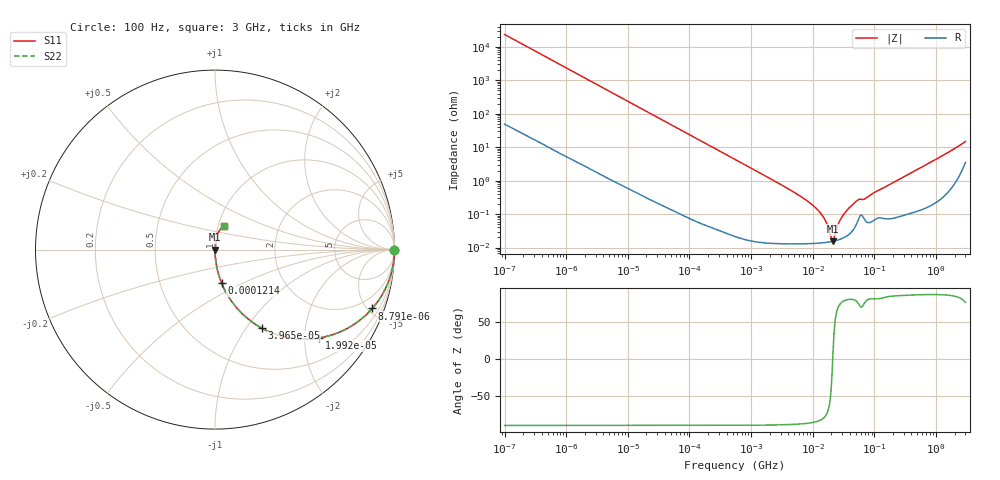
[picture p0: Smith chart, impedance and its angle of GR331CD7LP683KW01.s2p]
!Murata Part Number: GR331CD7LP683KW01
!These Parameters are Measured in Series Mode Connection
!Data Generated on Jan 08, 2026
!  o--ll--o
!Port1  Port2
!  o------o
!Operation Temp=25[degC], DC Bias Voltage=0[V]
!Freq. Start=100[Hz] Stop=3[GHz] 401[Steps]
# Hz S RI R 50
!Freq.(Hz) S11(Real) S11(Imag) S21(Real) S21(Imag) S12(Real) S12(Imag) S22(Real) S22(Imag)
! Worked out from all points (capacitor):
!   401 points, 100 Hz to 3 GHz, reference 50 ohm
!   read as one part in series: C = 68.2 nF near 109 Hz
!   lowest |Z| = 15.5 mohm at 21.25 MHz (marker M1)
!   series resonance near 21.1 MHz, so ESL is about 830 pH
!   S11 on the Smith chart (normalised r, x): 100 Hz: open; 8.791 kHz: 1.01, -5.34; 19.92 kHz: 1.01, -2.36; 39.66 kHz: 1.00, -1.19; 121.4 kHz: 1.00, -0.39; 3 GHz: 1.07, +0.28
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100  1 -0.00429  2.73e-05 0.00429  2.73e-05 0.00429  1 -0.00429
1788  0.994 -0.0759  0.00597 0.0759  0.00597 0.0759  0.994 -0.0759
8791  0.8763 -0.328  0.1237 0.328  0.1237 0.328  0.8763 -0.328
19917  0.5818 -0.492  0.4182 0.492  0.4182 0.492  0.5818 -0.492
31977  0.3514 -0.476  0.6486 0.476  0.6486 0.476  0.3514 -0.476
39655  0.2609 -0.4377  0.7391 0.4377  0.7391 0.4377  0.2609 -0.4377
66468  0.1122 -0.3142  0.8878 0.3142  0.8878 0.3142  0.1122 -0.3142
121426  0.0369 -0.1868  0.9631 0.1868  0.9631 0.1868  0.0369 -0.1868
547723  0.00207 -0.043  0.9979 0.043  0.9979 0.043  0.00207 -0.043
4141163  0.000159 -0.00549  0.9998 0.00549  0.9998 0.00549  0.000159 -0.00549
9794414  0.000135 -0.0019  0.9999 0.0019  0.9999 0.0019  0.000135 -0.0019
1.506283e7  0.00014 -0.000772  0.9999 0.000772  0.9999 0.000772  0.00014 -0.000772
1.713898e7  0.000144 -0.000471  0.9999 0.000471  0.9999 0.000471  0.000144 -0.000471
1.950129e7  0.00015 -0.000178  0.9999 0.000178  0.9999 0.000178  0.00015 -0.000178
2.12544e7  0.000154 1.66e-05  0.9998 -1.66e-05  0.9998 -1.66e-05  0.000154 1.66e-05
2.21892e7  0.000157 0.000114  0.9998 -0.000114  0.9998 -0.000114  0.000157 0.000114
2.999103e7  0.000188 0.000816  0.9998 -0.000816  0.9998 -0.000816  0.000188 0.000816
4.418008e7  0.000318 0.00189  0.9997 -0.00189  0.9997 -0.00189  0.000318 0.00189
5.478864e7  0.000683 0.00258  0.9993 -0.00258  0.9993 -0.00258  0.000683 0.00258
7.093284e7  0.000654 0.00282  0.9993 -0.00282  0.9993 -0.00282  0.000654 0.00282
1.751444e8  0.000776 0.00757  0.9992 -0.00757  0.9992 -0.00757  0.000776 0.00757
3e9  0.0516 0.1305  0.9484 -0.1305  0.9484 -0.1305  0.0516 0.1305
